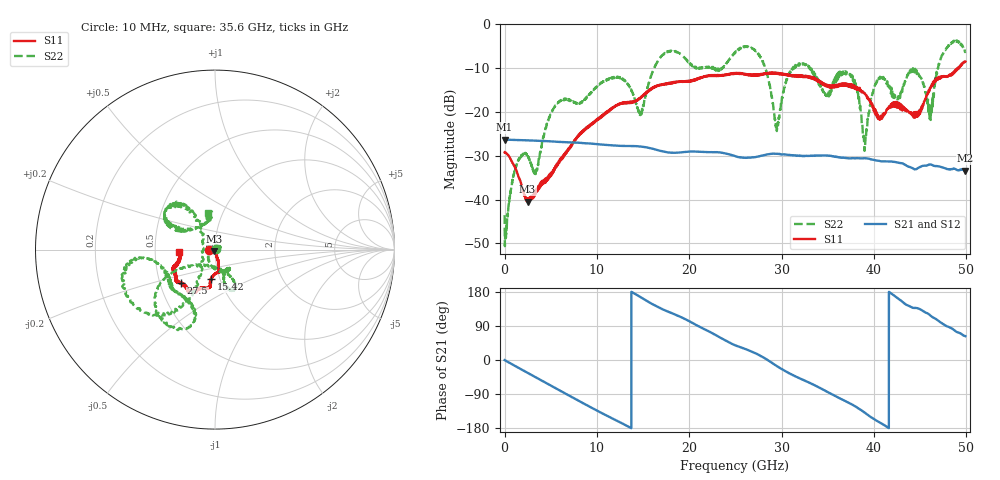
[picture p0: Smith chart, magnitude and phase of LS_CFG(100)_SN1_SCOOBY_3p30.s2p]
!Keysight Technologies,N5245B,MY58422026,A.13.80.08
!Date: Thursday, March 19, 2020 23:58:30
!Correction: S11(Full 2 Port(1,2))
!S21(Full 2 Port(1,2))
!S12(Full 2 Port(1,2))
!S22(Full 2 Port(1,2))
!S2P File: Measurements: S11, S21, S12, S22:
# Hz S DB R 50.0
!freq dBS11 angS11 dBS21 angS21 dBS12 angS12 dBS22 angS22
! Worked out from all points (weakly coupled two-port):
!   4991 points, 10 MHz to 49.91 GHz, reference 50 ohm
!   highest |S21| = -26.31 dB at 10 MHz (marker M1); lowest = -33.4 dB at 49.91 GHz (marker M2)
!   lowest |S11| = -40.5 dB at 2.5 GHz (marker M3), VSWR 1.02, Z = 49.4 - j0.74 ohm
!   |S11| at or under -10 dB: start of sweep to 49.12 GHz; 49.1741 GHz to 49.22035 GHz (46.25 MHz wide, 0.094 % of centre)
!   |S22| runs from -50.6 to -3.7 dB; largest |S21 - S12| = 0.00044
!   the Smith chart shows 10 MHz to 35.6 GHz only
!   S11 on the Smith chart (normalised r, x): 10 MHz: 0.93, -0.00; 15.42 GHz: 0.91, -0.31; 27.5 GHz: 0.64, -0.26; 35.6 GHz: 0.67, -0.02
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1e7  -29.24 -175.6  -26.31 -0.2  -26.31 -0.3  -43.56 7.7
1.29e9  -33.31 -173.1  -26.41 -17.6  -26.41 -17.6  -32.19 -18.4
2.5e9  -40.47 -127.8  -26.51 -33.9  -26.50 -33.9  -30.06 44.4
5.75e9  -31.72 -69.7  -26.84 -77.6  -26.83 -77.6  -17.97 -77.0
8.33e9  -24.90 -74.9  -27.10 -111.7  -27.09 -111.6  -17.80 -62.5
1.542e10  -15.62 -96.8  -28.11 155.8  -28.11 156.0  -15.21 -148.3
1.665e10  -14.04 -97.7  -28.77 139.2  -28.76 139.3  -8.24 -145.4
1.985e10  -13.01 -104.6  -29.09 104.4  -29.08 104.5  -8.59 -106.5
2.496e10  -11.30 -123.5  -30.08 39.1  -30.06 39.3  -6.55 -171.1
2.75e10  -11.52 -135.2  -30.17 13.9  -30.18 14.2  -6.69 -127.7
2.947e10  -11.09 -140.9  -29.57 -15.6  -29.56 -15.3  -23.51 -176.4
3.103e10  -11.64 -148.1  -29.88 -37.5  -29.89 -37.2  -10.42 125.5
3.328e10  -12.20 -158.6  -30.01 -63.2  -30.02 -62.7  -10.65 153.1
3.56e10  -13.99 -176.3  -30.17 -92.7  -30.11 -92.2  -13.97 101.3
3.769e10  -14.50 174.3  -30.58 -118.3  -30.52 -118.4  -11.97 130.7
3.902e10  -15.83 170.0  -30.57 -139.1  -30.55 -139.3  -28.16 -113.9
4.021e10  -20.64 157.1  -31.06 -158.9  -31.03 -159.0  -13.48 -9.1
4.16e10  -18.87 104.9  -31.31 -179.6  -31.34 -179.6  -14.20 22.4
4.445e10  -20.56 54.0  -33.11 137.3  -33.14 137.6  -10.42 -17.0
4.614e10  -14.42 8.3  -32.00 116.9  -32.02 117.1  -21.53 -50.9
4.757e10  -11.86 7.5  -32.78 93.6  -32.79 93.8  -6.29 -80.3
4.991e10  -8.54 -12.6  -33.40 63.1  -33.42 63.2  -6.28 -28.6
